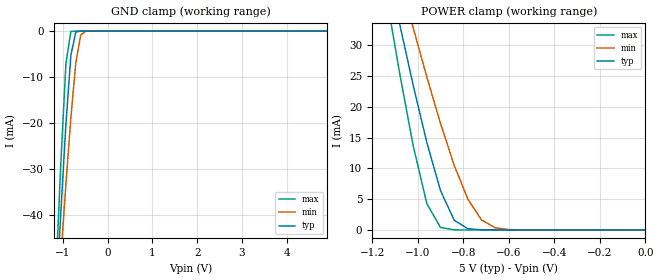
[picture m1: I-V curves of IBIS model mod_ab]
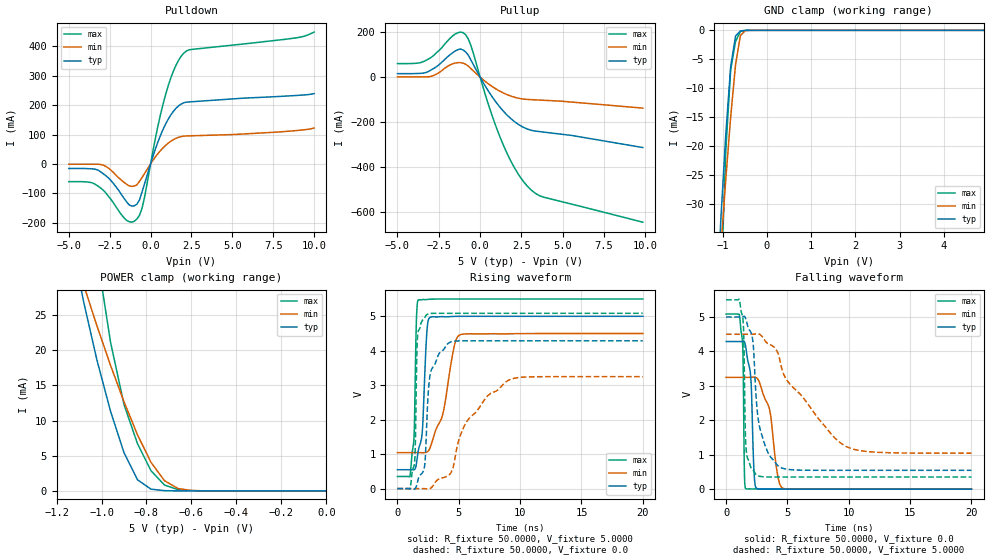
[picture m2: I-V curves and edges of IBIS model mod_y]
| IBIS (I/O, Buffer, Information, Specification) Model, officially
| electronic behavioral standard for Buffer structures of digital pins.
[IBIS ver]  4.0
[File name] 54act32_5v_rev1.ibs
[File Rev]  1.0
[Date]   7 May 2018
[Source]   CAD & Design Services (Catania) - STMicroelectronics
[Notes]
   (Note1)  This IBIS model is the model of the product with package
   (Flat-14);
   (Note2)  This IBIS model is extracted with nominal 5V power supply
   (min:4.5V, typ:5.0V, max:5.5V);
   (Note3)  This IBIS model has some Notes about the non-monotonicity
   of the I-V curves, but they are not indicative of problems
   inside the model;
[Disclaimer]
   Customers are solely responsible for all aspects of their
   own product designs or applications using this IBIS Model.
   STMicroelectronics assumes no liability for Custmer Designs
   and applications associated to this IBIS Model.
   In the use of this IBIS Model Customer shall not modify,
   disassemble, alter this Model in whole or in part.
   If Customers do not accept these terms, the IBIS Model
   may not be used. For any problems or modifications please
   contact STMicroelectronics (www.st.com).
[Copyright] (c) 2018 STMicroelectronics
|   Component 54ACT32
[Component] 54ACT32
[Manufacturer] STMicroelectronics
[Package]
| variable   typ   min   max
R_pkg   0.0   0.0   0.0
L_pkg   0.0H   0.0H   0.0H
C_pkg   0.0F   0.0F   0.0F
[Pin]   signal_name   model_name   R_pin   L_pin   C_pin
1   1A   mod_ab   78.8m   2.61nH   1.01pF
2   1B   mod_ab   34.7m   0.86nH   0.80pF
3   1Y   mod_y   26.6m   0.75nH   1.04pF
4   2A   mod_ab   26.6m   0.75nH   1.04pF
5   2B   mod_ab   26.6m   0.75nH   1.04pF
6   2Y   mod_y   34.7m   0.86nH   0.80pF
7   GND   GND   78.8m   2.61nH   1.01pF
8   3Y   mod_y   78.8m   2.61nH   1.01pF
9   3A   mod_ab   34.7m   0.86nH   0.80pF
10   3B   mod_ab   26.6m   0.75nH   1.04pF
11   4Y   mod_y   26.6m   0.75nH   1.04pF
12   4A   mod_ab   26.6m   0.75nH   1.04pF
13   4B   mod_ab   34.7m   0.86nH   0.80pF
14   VCC   POWER   78.8m   2.61nH   1.01pF
| Models and submodels in the file (2): mod_ab (Input), mod_y (I/O)
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|   Model mod_ab
[Model]   mod_ab
Model_type Input
Vinl  =   1.500V
Vinh  =   3.500V
C_comp   0.532pF   0.386pF   0.702pF
[Temperature Range]  25.0000   0.1250k   -55.0000
[Voltage Range]   5.0000V   4.5000V   5.5000V
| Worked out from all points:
|   GND clamp passes 1 mA (typ) near -0.73 V on its own axis
|   POWER clamp passes 1 mA (typ) near -0.81 V on its own axis
[GND_clamp]
|Voltage   I(typ)   I(min)   I(max)
-5V       -806.2mA   -661.5mA   -989mA
-1.15V    -58.36mA   -64.46mA   -52.14mA
-1.04V    -38.69mA   -48.58mA   -27.89mA
-930mV    -20.24mA   -33.23mA   -7.088mA
-820mV    -5.298mA   -18.88mA   -92.01uA
-710mV    -199.8uA   -6.915mA   -269.8nA
-600mV    -2.871uA   -855.1uA   -789.3pA
-490mV    -39.72nA   -40.25uA   -15.19pA
4.9V      9.6pA      196.2nA    8.6pA
[POWER_clamp]
|Voltage   I(typ)   I(min)   I(max)
-4.98V    788.6mA    643.8mA    971.6mA
-1.14V    44.05mA    49.59mA    38.51mA
-1.08V    33.57mA    41.11mA    25.59mA
-1.02V    23.51mA    32.83mA    13.69mA
-960mV    14.21mA    24.84mA    4.274mA
-900mV    6.4mA      17.31mA    404.4uA
-840mV    1.595mA    10.51mA    18.06uA
-780mV    203uA      5.024mA    745.1nA
-720mV    20.37uA    1.632mA    30.64nA
-660mV    1.978uA    359uA      1.272nA
-600mV    191.5nA    65.93uA    65.13pA
0V        10pA       55.89pA    11pA
|   Model mod_y
[Model]   mod_y
Model_type I/O
Polarity   Non-Inverting
Vinl  =   1.500V
Vinh  =   3.500V
Vmeas =   2.500V
C_comp   2.925pF   2.219pF   3.682pF
[Temperature Range]  25.0000   0.1250k   -55.0000
[Voltage Range]   5.0000V   4.5000V   5.5000V
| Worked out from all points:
|   slope of the pulldown table from 0 to 0.75 V, typ, clamps not added: 6.47 ohm
|   slope of the pullup table from 0 to 0.75 V, typ, clamps not added: 8.35 ohm
|   GND clamp passes 1 mA (typ) near -0.71 V on its own axis
|   POWER clamp passes 1 mA (typ) near -0.81 V on its own axis
|   rising waveform, R_fixture 50.0000, V_fixture 5.0000: 20-80 % time 373ps typ, 1.29ns min, 185ps max; typ from 0.548 V to 5 V
|   rising waveform, R_fixture 50.0000, V_fixture 0.0: 20-80 % time 489ps typ, 2.57ns min, 153ps max; typ from 0 V to 4.29 V
|   falling waveform, R_fixture 50.0000, V_fixture 0.0: 20-80 % time 274ps typ, 889ps min, 106ps max; typ from 4.29 V to 0 V
|   falling waveform, R_fixture 50.0000, V_fixture 5.0000: 20-80 % time 799ps typ, 3.92ns min, 157ps max; typ from 5 V to 0.548 V
[Pulldown]
|Voltage   I(typ)   I(min)   I(max)
-5V       -15.45mA   -1.023mA   -60.15mA
-3.24V    -20.45mA   -1.023mA   -74.2mA
-2.44V    -55.33mA   -20.13mA   -119.2mA
-1.48V    -127.5mA   -68.36mA   -191.5mA
-1V       -142.4mA   -75.29mA   -195.1mA
-680mV    -122.5mA   -59.31mA   -175mA
-520mV    -94.67mA   -46.04mA   -150.4mA
440mV     73.46mA    34.38mA    126.4mA
920mV     135.7mA    63.13mA    236mA
1.4V      179.2mA    82.74mA    316.2mA
2.04V     208.1mA    94.66mA    377.2mA
10V       239.2mA    122mA      448.2mA
[Pullup]
|Voltage   I(typ)   I(min)   I(max)
-5V       15.45mA    1.023mA    60.15mA
-3.44V    17.65mA    1.023mA    68.55mA
-2.8V     38.74mA    7.798mA    97.13mA
-1.52V    115.8mA    62.33mA    191mA
-1.04V    121.2mA    62.27mA    198mA
-560mV    76.32mA    38.03mA    141.1mA
560mV     -69.07mA   -33.2mA    -135.3mA
1.36V     -147.6mA   -69.01mA   -294.6mA
2.16V     -202.5mA   -91.16mA   -413.9mA
2.96V     -233.7mA   -99.72mA   -493.1mA
3.76V     -243.9mA   -102.8mA   -532.4mA
9.84V     -313.3mA   -137.9mA   -645.4mA
[GND_clamp]
|Voltage   I(typ)   I(min)   I(max)
-5V       -952.3mA   -788.1mA   -1.129A
-1.15V    -49.18mA   -49.48mA   -71.61mA
-1.04V    -32.37mA   -37.34mA   -44.71mA
-930mV    -17.97mA   -25.74mA   -20.77mA
-820mV    -6.299mA   -14.99mA   -6.821mA
-710mV    -992.3uA   -5.948mA   -1.936mA
-600mV    -109.4uA   -900.4uA   -197.5uA
-490mV    -9.5uA     -57.98uA   -7.173uA
-380mV    -722.1nA   -4.418uA   -236.7nA
4.9V      105.2pA    213.3nA    21.77pA
[POWER_clamp]
|Voltage   I(typ)   I(min)   I(max)
-4.98V    938.8mA    774mA      1.116A
-1.14V    36.56mA    35.49mA    62.12mA
-1.08V    26.96mA    29.34mA    47.45mA
-1.02V    18.56mA    23.44mA    33.53mA
-960mV    11.34mA    17.86mA    21.17mA
-900mV    5.438mA    12.67mA    12.28mA
-840mV    1.583mA    7.976mA    6.708mA
-780mV    254.1uA    4.066mA    2.871mA
-720mV    36.76uA    1.453mA    835.5uA
-660mV    6.645uA    343.8uA    185.6uA
-600mV    1.494uA    64.84uA    37.53uA
0V        111.1pA    2.989nA    31.8pA
[Ramp]
| variable   typ   min   max
dV/dt_r   2.5731/0.6097n   1.9495/2.6788n   3.0520/0.4368n
dV/dt_f   2.6711/0.8652n   2.0730/3.9545n   3.0889/0.4272n
R_load = 50.0000
[Rising Waveform]
R_fixture= 50.0000
V_fixture= 5.0000
V_fixture_min= 4.5000
V_fixture_max= 5.5000
|time   V(typ)   V(min)   V(max)
0s        547.7mV    1.045V     351.6mV
1.04ns    547.9mV    1.045V     392mV
1.34ns    544.6mV    1.045V     1.417V
1.54ns    711.5mV    1.045V     4.841V
1.7ns     1.106V     1.045V     5.475V
2.02ns    1.626V     1.041V     5.484V
2.38ns    4.46V      1.057V     5.486V
2.66ns    4.971V     1.185V     5.497V
5.04ns    4.999V     4.453V     5.5V
20ns      5V         4.5V       5.5V
[Rising Waveform]
R_fixture= 50.0000
V_fixture= 0.0
V_fixture_min= 0.0
V_fixture_max= 0.0
|time   V(typ)   V(min)   V(max)
0s        145.2pV    0V         93.97pV
1.38ns    -13.06mV   -41.47uV   696.7mV
1.64ns    196mV      150.1uV    4.446V
2.2ns     624.3mV    -2.049mV   4.935V
2.4ns     1.991V     -8.382mV   5.049V
2.72ns    3.394V     14.7mV     5.083V
4.36ns    4.257V     456.6mV    5.087V
5.68ns    4.288V     1.962V     5.087V
9.04ns    4.288V     3.144V     5.087V
20ns      4.288V     3.248V     5.087V
[Falling Waveform]
R_fixture= 50.0000
V_fixture= 0.0
V_fixture_min= 0.0
V_fixture_max= 0.0
|time   V(typ)   V(min)   V(max)
0s        4.288V     3.248V     5.087V
1.32ns    4.29V      3.248V     4.355V
1.38ns    4.296V     3.248V     3.813V
1.5ns     4.278V     3.248V     342.4mV
1.6ns     4.133V     3.248V     15.58mV
2ns       3.282V     3.248V     7.378mV
2.28ns    473.8mV    3.254V     8.254mV
2.52ns    14.03mV    3.226V     5.304mV
4.52ns    2.901mV    48.87mV    11.94uV
20ns      -76.39nV   1.182uV    -116.8nV
[Falling Waveform]
R_fixture= 50.0000
V_fixture= 5.0000
V_fixture_min= 4.5000
V_fixture_max= 5.5000
|time   V(typ)   V(min)   V(max)
0s        5V         4.5V       5.5V
1.34ns    5.002V     4.5V       5.035V
1.42ns    5.016V     4.5V       4.677V
1.54ns    5.001V     4.5V       2.073V
1.66ns    4.878V     4.5V       1.045V
2.18ns    4.296V     4.5V       550.5mV
2.5ns     2.413V     4.516V     408.7mV
4.3ns     659.5mV    3.866V     351.7mV
9.7ns     547.7mV    1.254V     351.6mV
20ns      547.7mV    1.045V     351.6mV
